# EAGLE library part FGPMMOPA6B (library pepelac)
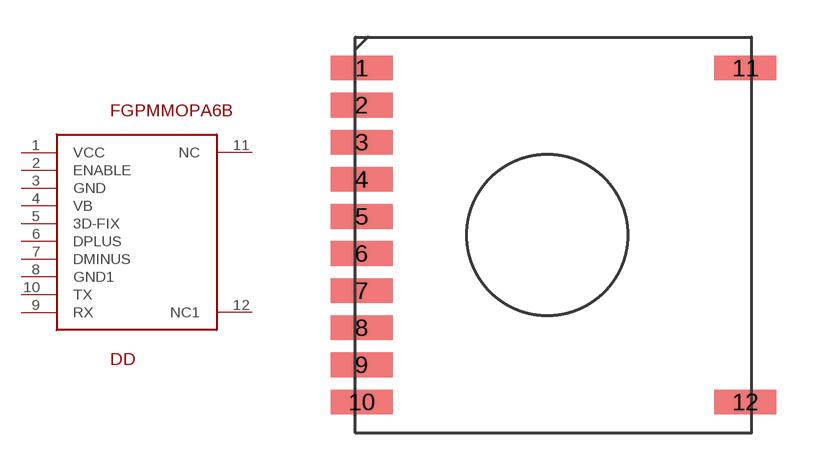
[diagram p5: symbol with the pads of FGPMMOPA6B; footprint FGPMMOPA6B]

Designator prefix DD

## FGPMMOPA6B  [FGPMMOPA6B]
1  VCC
2  ENABLE
3  GND
4  VB
5  3D-FIX
6  DPLUS
7  DMINUS
8  GND1
9  RX
10  TX
11  NC
12  NC1

## Footprint FGPMMOPA6B (pad centres in mm)
smd 2.5 x 1: 1 -7.5,6.75; 2 -7.5,5.25; 3 -7.5,3.75; 4 -7.5,2.25; 5 -7.5,0.75; 6 -7.5,-0.75; 7 -7.5,-2.25; 8 -7.5,-3.75; 9 -7.5,-5.25; 10 -7.5,-6.75; 11 8,6.75; 12 8,-6.75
